|   TEXAS INSTRUMENTS INCORPORATED
|   Standard Linear and Logic
|   IBIS Model of SN74ALVCH162268
|   12 BIT TO 24 BIT REGISTERED BUS EXCHANGER
|   TSSOP 56 pin package(DGG)
|   SSOP 56 pin package(DL)
[IBIS Ver]   3.2
[Comment char]   |_char
[File Name]   alvch162268.ibs
[File Rev]   1.0
[Date]   07-26-2000
[Source]   File originated at Texas Instruments Incorporated
[Notes]   The following is an IBIS list for SN74ALVCH162268.
   - All test data contained in this file are derived from hspice
   (tm) simulations.
   - File created by Md Sagir Hasnain, SLL applications.
|   -For Questions or Comments please mailto:sllibis@ti.com
|*   Property of Texas Instruments Incorporated.  Unauthorized   *
|*   reproduction and/or distribution is strictly prohibited.   *
|*   This product is protected under copyright law.   *
|*   Created 1998, (C) Copyright 1998,   *
|*   Texas Instruments Incorporated   *
|*   All Rights Reserved   *
|*   UNLESS THERE IS A SIGNED, WRITTEN AGREEMENT TO THE   *
|*   CONTRARY, TEXAS INSTRUMENTS ("TI") IS PROVIDING THE SPICE   *
|*   MODELS "AS IS" AND WITHOUT ANY WARRANTY, EXPRESSED OR   *
|*   IMPLIED.  TI assumes no liability for:   *
|*   1) the accuracy of the IBIS models provided to your   *
|*   company;   *
|*   2) the proper functioning of these IBIS models in your   *
|*   design or for any resulting applications; or   *
|*   3) infringement of patents, copyrights or intellectual   *
|*   property rights resulting from your use of these   *
|*   IBIS models.   *
|*   TI provides IBIS Models as a service to our customers.   *
|*   You and your company shall not distribute, sell or give   *
|*   these models to anyone else without prior written   *
|*   permission from TI.   *
|*   TI reserves the right to make changes to our products or   *
|*   to discontinue any semiconductor product or service   *
|*   without notice, and advises our customers to obtain the   *
|*   latest version of relevant information to verify, before   *
|*   placing orders, that the information being relied on is   *
|*   current.   *
|*   Please be aware that your receipt and use of the IBIS   *
|*   information provided shall serve as acceptance of these   *
|*   terms and conditions.  If you do not accept these terms,   *
|*   you should return or destroy the IBIS models and any   *
|*   other accompanying information immediately.   *
|   TSSOP PACKAGE (DGG)
[Component]   ALVCH162268_DGG
[manufacturer]   Texas Instruments Incorporated.
[Package]
|   typ   min   max
R_pkg   0.045   0.035   0.062
L_pkg   3.324nH   2.403nH   5.094nH
C_pkg   0.564pF   0.341pF   0.914nH
[Pin]   signal_name   model_name   R_pin   L_pin   C_pin
1   OEA_BAR   ALVCH162268_IN1   0.062   5.094nH   0.856pF
2   CLKEN1B_BAR   ALVCH162268_IN1   0.061   4.621nH   0.902pF
3   2B3   ALVCH162268_I_O_B   0.06   4.316nH   0.802pF
4   GND   GND   0.059   3.968nH   0.698pF
5   2B2   ALVCH162268_I_O_B   0.057   3.716nH   0.649pF
6   2B1   ALVCH162268_I_O_B   0.042   3.517nH   0.652pF
7   VCC   POWER   0.041   3.16nH   0.57pF
8   A1   ALVCH162268_I_O_A   0.039   2.981nH   0.482pF
9   A2   ALVCH162268_I_O_A   0.039   2.809nH   0.447pF
10   A3   ALVCH162268_I_O_A   0.038   2.715nH   0.409pF
11   GND   GND   0.041   2.675nH   0.391pF
12   A4   ALVCH162268_I_O_A   0.039   2.536nH   0.366pF
13   A5   ALVCH162268_I_O_A   0.039   2.457nH   0.348pF
14   A6   ALVCH162268_I_O_A   0.038   2.411nH   0.353pF
15   A7   ALVCH162268_I_O_A   0.039   2.456nH   0.355pF
16   A8   ALVCH162268_I_O_A   0.039   2.471nH   0.349pF
17   A9   ALVCH162268_I_O_A   0.04   2.58nH   0.37pF
18   GND   GND   0.038   2.651nH   0.389pF
19   A10   ALVCH162268_I_O_A   0.038   2.739nH   0.411pF
20   A11   ALVCH162268_I_O_A   0.039   2.838nH   0.449pF
21   A12   ALVCH162268_I_O_A   0.038   2.988nH   0.484pF
22   VCC   POWER   0.038   3.105nH   0.564pF
23   1B1   ALVCH162268_I_O_B   0.04   3.427nH   0.638pF
24   1B2   ALVCH162268_I_O_B   0.056   3.654nH   0.641pF
25   GND   GND   0.057   3.932nH   0.7pF
26   1B3   ALVCH162268_I_O_B   0.058   4.257nH   0.806pF
27   CLKEN2B_BAR   ALVCH162268_IN1   0.057   4.58nH   0.914pF
28   SEL_BAR   ALVCH162268_SEL   0.059   5.038nH   0.861pF
29   CLK   ALVCH162268_CLK   0.06   5.058nH   0.858pF
30   CLKENA1_BAR   ALVCH162268_IN1   0.056   4.543nH   0.904pF
31   1B4   ALVCH162268_I_O_B   0.057   4.24nH   0.803pF
32   GND   GND   0.057   3.929nH   0.7pF
33   1B5   ALVCH162268_I_O_B   0.056   3.616nH   0.637pF
34   1B6   ALVCH162268_I_O_B   0.037   3.368nH   0.64pF
35   VCC   POWER   0.036   3.024nH   0.563pF
36   1B7   ALVCH162268_I_O_B   0.035   2.876nH   0.474pF
37   1B8   ALVCH162268_I_O_B   0.035   2.745nH   0.444pF
38   1B9   ALVCH162268_I_O_B   0.037   2.683nH   0.405pF
39   GND   GND   0.038   2.603nH   0.382pF
40   1B10   ALVCH162268_I_O_B   0.038   2.51nH   0.362pF
41   1B11   ALVCH162268_I_O_B   0.036   2.412nH   0.341pF
42   1B12   ALVCH162268_I_O_B   0.038   2.416nH   0.349pF
43   2B12   ALVCH162268_I_O_B   0.037   2.403nH   0.349pF
44   2B111   ALVCH162268_I_O_B   0.037   2.429nH   0.341pF
45   2B10   ALVCH162268_I_O_B   0.036   2.482nH   0.358pF
46   GND   GND   0.037   2.615nH   0.381pF
47   2B9   ALVCH162268_I_O_B   0.035   2.669nH   0.402pF
48   2B8   ALVCH162268_I_O_B   0.036   2.763nH   0.442pF
49   2B7   ALVCH162268_I_O_B   0.036   2.942nH   0.478pF
50   VCC   POWER   0.035   3.053nH   0.564pF
51   2B6   ALVCH162268_I_O_B   0.036   3.409nH   0.641pF
52   2B5   ALVCH162268_I_O_B   0.058   3.698nH   0.641pF
53   GND   GND   0.059   3.975nH   0.697pF
54   2B4   ALVCH162268_I_O_B   0.061   4.327nH   0.802pF
55   CLKENA2_BAR   ALVCH162268_IN1   0.061   4.624nH   0.905pF
56   OEB_BAR   ALVCH162268_IN1   0.06   5.063nH   0.858pF
|   SSOP PACKAGE (DL)
[Component]   ALVCH162268_DL
[manufacturer]   Texas Instruments Incorporated.
[Package]
|   typ   min   max
R_pkg   0.055   0.048   0.067
L_pkg   6.539nH   4.802nH   9.746nH
C_pkg   0.85pF   0.5pF   1.351pF
[Pin]   signal_name   model_name   R_pin   L_pin   C_pin
1   OEA_BAR   ALVCH162268_IN1   0.064   9.646nH   1.202pF
2   CLKEN1B_BAR   ALVCH162268_IN1   0.059   8.723nH   1.348pF
3   2B3   ALVCH162268_I_O_B   0.059   8.139nH   1.223pF
4   GND   GND   0.056   7.554nH   1.088pF
5   2B2   ALVCH162268_I_O_B   0.054   6.991nH   0.966pF
6   2B1   ALVCH162268_I_O_B   0.053   6.659nH   0.973pF
7   VCC   POWER   0.055   6.321nH   0.905pF
8   A1   ALVCH162268_I_O_A   0.055   5.942nH   0.713pF
9   A2   ALVCH162268_I_O_A   0.057   5.767nH   0.678pF
10   A3   ALVCH162268_I_O_A   0.054   5.459nH   0.631pF
11   GND   GND   0.051   5.224nH   0.638pF
12   A4   ALVCH162268_I_O_A   0.048   5.088nH   0.601pF
13   A5   ALVCH162268_I_O_A   0.05   5.021nH   0.518pF
14   A6   ALVCH162268_I_O_A   0.051   4.802nH   0.5pF
15   A7   ALVCH162268_I_O_A   0.051   4.803nH   0.5pF
16   A8   ALVCH162268_I_O_A   0.05   5.021nH   0.518pF
17   A9   ALVCH162268_I_O_A   0.048   5.088nH   0.601pF
18   GND   GND   0.051   5.224nH   0.638pF
19   A10   ALVCH162268_I_O_A   0.054   5.459nH   0.631pF
20   A11   ALVCH162268_I_O_A   0.057   5.768nH   0.677pF
21   A12   ALVCH162268_I_O_A   0.055   5.942nH   0.715pF
22   VCC   POWER   0.055   6.321nH   0.907pF
23   1B1   ALVCH162268_I_O_B   0.053   6.659nH   0.972pF
24   1B2   ALVCH162268_I_O_B   0.054   6.991nH   0.966pF
25   GND   GND   0.056   7.554nH   1.087pF
26   1B3   ALVCH162268_I_O_B   0.059   8.139nH   1.223pF
27   CLKEN2B_BAR   ALVCH162268_IN1   0.059   8.727nH   1.351pF
28   SEL_BAR   ALVCH162268_SEL   0.067   9.746nH   1.21pF
29   CLK   ALVCH162268_CLK   0.063   9.63nH   1.203pF
30   CLKENA1_BAR   ALVCH162268_IN1   0.06   8.751nH   1.349pF
31   1B4   ALVCH162268_I_O_B   0.06   8.184nH   1.224pF
32   GND   GND   0.056   7.543nH   1.087pF
33   1B5   ALVCH162268_I_O_B   0.054   7.005nH   0.969pF
34   1B6   ALVCH162268_I_O_B   0.056   6.714nH   0.975pF
35   VCC   POWER   0.058   6.384nH   0.909pF
36   1B7   ALVCH162268_I_O_B   0.057   5.976nH   0.717pF
37   1B8   ALVCH162268_I_O_B   0.057   5.743nH   0.677pF
38   1B9   ALVCH162268_I_O_B   0.055   5.469nH   0.631pF
39   GND   GND   0.055   5.328nH   0.644pF
40   1B10   ALVCH162268_I_O_B   0.052   5.189nH   0.606pF
41   1B11   ALVCH162268_I_O_B   0.052   5.053nH   0.519pF
42   1B12   ALVCH162268_I_O_B   0.052   4.825nH   0.502pF
43   2B12   ALVCH162268_I_O_B   0.054   4.896nH   0.506pF
44   2B111   ALVCH162268_I_O_B   0.052   5.093nH   0.521pF
45   2B10   ALVCH162268_I_O_B   0.051   5.179nH   0.608pF
46   GND   GND   0.054   5.314nH   0.645pF
47   2B9   ALVCH162268_I_O_B   0.055   5.511nH   0.632pF
48   2B8   ALVCH162268_I_O_B   0.057   5.77nH   0.677pF
49   2B7   ALVCH162268_I_O_B   0.055   5.956nH   0.716pF
50   VCC   POWER   0.055   6.32nH   0.905pF
51   2B6   ALVCH162268_I_O_B   0.052   6.621nH   0.968pF
52   2B5   ALVCH162268_I_O_B   0.053   6.974nH   0.966pF
53   GND   GND   0.057   7.571nH   1.089pF
54   2B4   ALVCH162268_I_O_B   0.057   8.097nH   1.219pF
55   CLKENA2_BAR   ALVCH162268_IN1   0.059   8.723nH   1.349pF
56   OEB_BAR   ALVCH162268_IN1   0.061   9.56nH   1.199pF
|   Model ALVCH162268 OUTPUT model
[Model Selector]   ALVCH162268_I_O_B
ALVCH162268_I_O_B_33 3.3v
ALVCH162268_I_O_B_25 2.5v
|   Model ALVCH162268 OUTPUT model
[Model Selector]   ALVCH162268_I_O_A
ALVCH162268_I_O_A_33 3.3v
ALVCH162268_I_O_A_25 2.5v
|   ALVCH162268 Input (IN1) model
[Model Selector]   ALVCH162268_IN1
ALVCH162268_IN1_33 3.3v
ALVCH162268_IN1_25 2.5v
|   ALVCH162268 Input (SEL) model
[Model Selector]   ALVCH162268_SEL
ALVCH162268_SEL_33 3.3v
ALVCH162268_SEL_25 2.5v
|   ALVCH162268 Input (CLK) model
[Model Selector]   ALVCH162268_CLK
ALVCH162268_CLK_33 3.3v
ALVCH162268_CLK_25 2.5v
| Models and submodels in the file (10): ALVCH162268_I_O_B_33 (I/O), ALVCH162268_I_O_B_25 (I/O), ALVCH162268_I_O_A_33 (I/O), ALVCH162268_I_O_A_25 (I/O), ALVCH162268_IN1_33 (Input), ALVCH162268_IN1_25 (Input), ALVCH162268_SEL_33 (Input), ALVCH162268_SEL_25 (Input), ALVCH162268_CLK_33 (Input), ALVCH162268_CLK_25 (Input)
